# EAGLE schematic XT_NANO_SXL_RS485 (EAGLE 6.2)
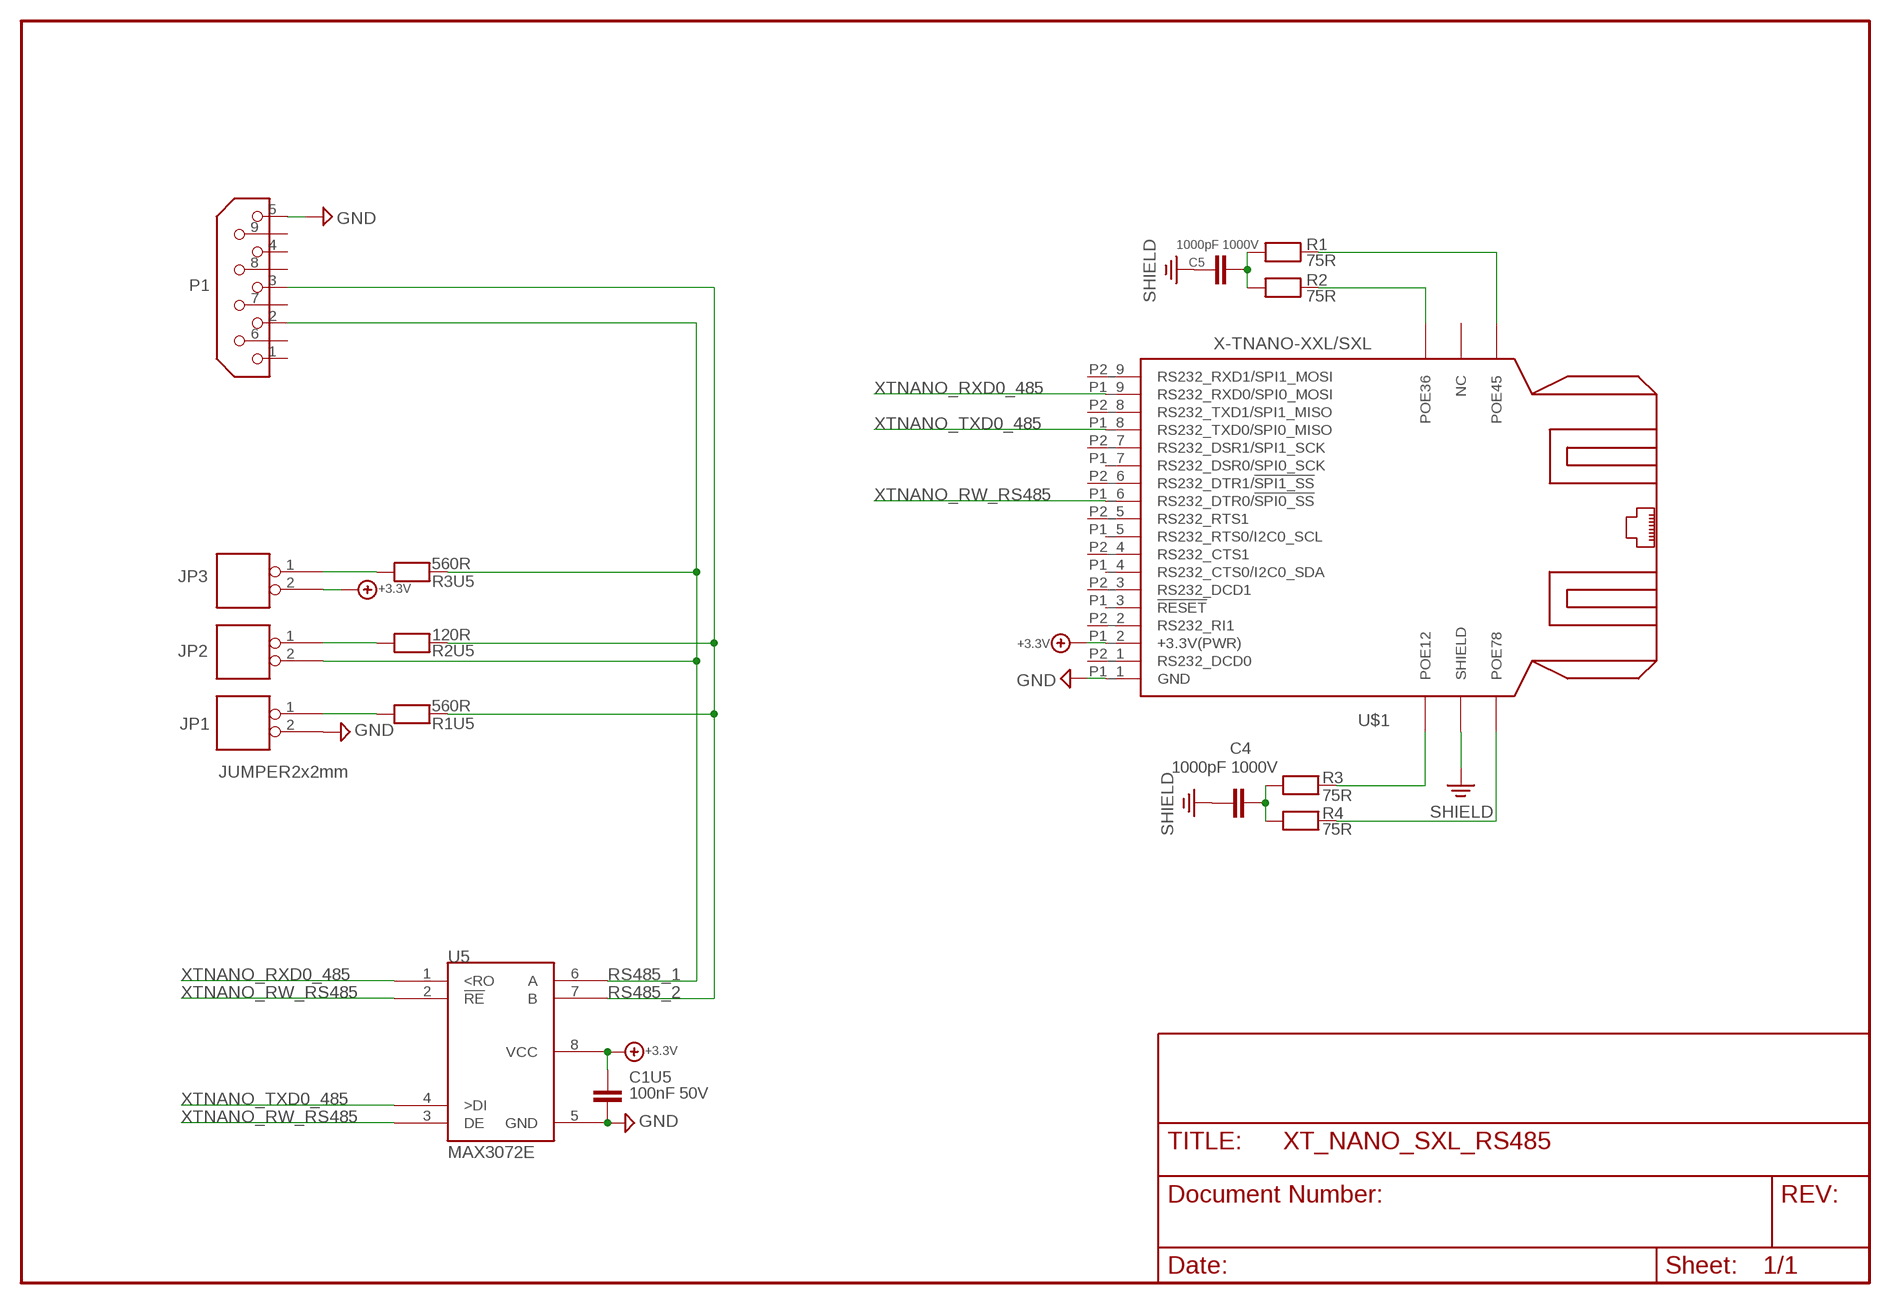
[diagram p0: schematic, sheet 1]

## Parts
C1U5  100nF 50V  CHIP-C-0603  [SMD-0603]
C4  1000pF 1000V  CHIP-C-1210  [SMD-1210]
C5  1000pF 1000V  CHIP-C-1210  [SMD-1210]
JP1  JUMPER2x2mm  JP2  [ROLF_SQW1X2]
JP2  JUMPER2x2mm  JP2  [ROLF_SQW1X2]
JP3  JUMPER2x2mm  JP2  [ROLF_SQW1X2]
P1  DB9  [MSUB9-5]
R1  75R  CHIP-R-0603  [SMD-0603]
R1U5  560R  CHIP-R-0603  [SMD-0603]
R2  75R  CHIP-R-0603  [SMD-0603]
R2U5  120R  CHIP-R-0603  [SMD-0603]
R3  75R  CHIP-R-0603  [SMD-0603]
R3U5  560R  CHIP-R-0603  [SMD-0603]
R4  75R  CHIP-R-0603  [SMD-0603]
U5  MAX3072E  MAX3072E_SO8  [SO-8]
U$1  X-TNANO-XXL/SXL  [XT-NANO-XXL/SXL]

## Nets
+3.3V: C1U5.2 JP3.2 U5.8(VCC) U$1.P1_2(+3.3V(PWR))
GND: C1U5.1 JP1.2 P1.5 U5.5(GND) U$1.P1_1(GND)
N14469550: JP2.1 R2U5.2
N15158340: JP1.1 R1U5.2
N15158360: JP3.1 R3U5.2
N$1: C5.1 R1.1 R2.1
N$2: C4.2 R3.1 R4.1
N$4: R2.2 U$1.POE36
N$6: R1.2 U$1.POE45
N$20: R3.2 U$1.POE12
N$21: R4.2 U$1.POE78
RS485_1: JP2.2 P1.2 R3U5.1 U5.6(A)
RS485_2: P1.3 R1U5.1 R2U5.1 U5.7(B)
SHIELD: C4.1 C5.2 U$1.SHIELD
XTNANO_RW_RS485: U5.2(!RE) U5.3(DE) U$1.P1_6(RS232_DTR0/!SPI0_SS!)
XTNANO_RXD0_485: U5.1(<RO) U$1.P1_9(RS232_RXD0/SPI0_MOSI)
XTNANO_TXD0_485: U5.4(>DI) U$1.P1_8(RS232_TXD0/SPI0_MISO)
Unconnected: P1.1 P1.4 P1.6 P1.7 P1.8 P1.9 U$1.FLASH(NC) U$1.P1_3(!RESET) U$1.P1_4(RS232_CTS0/I2C0_SDA) U$1.P1_5(RS232_RTS0/I2C0_SCL) U$1.P1_7(RS232_DSR0/SPI0_SCK) U$1.P2_1(RS232_DCD0) U$1.P2_2(RS232_RI1) U$1.P2_3(RS232_DCD1) U$1.P2_4(RS232_CTS1) U$1.P2_5(RS232_RTS1) U$1.P2_6(RS232_DTR1/!SPI1_SS!) U$1.P2_7(RS232_DSR1/SPI1_SCK) U$1.P2_8(RS232_TXD1/SPI1_MISO) U$1.P2_9(RS232_RXD1/SPI1_MOSI)

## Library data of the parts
C1U5 = mea-lib:CHIP-C-?: Chip capacitance
C4 C5 = XTMACRO:CHIP-C-?: Chip capacitance
JP1-JP3 = XTMACRO_AS:JP2
P1 = XTMACRO:DB9
R1-R4 = XTMACRO:CHIP-R-?: Chip resistors
R1U5 R2U5 R3U5 = mea-lib:CHIP-R-?: Chip resistors
U5 = XTMACRO_AS:MAX3072E_SO8
U$1 = ak-devices:X-TNANO-XXL/SXL: AK-NORD XT-NANO-XXL/SXL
